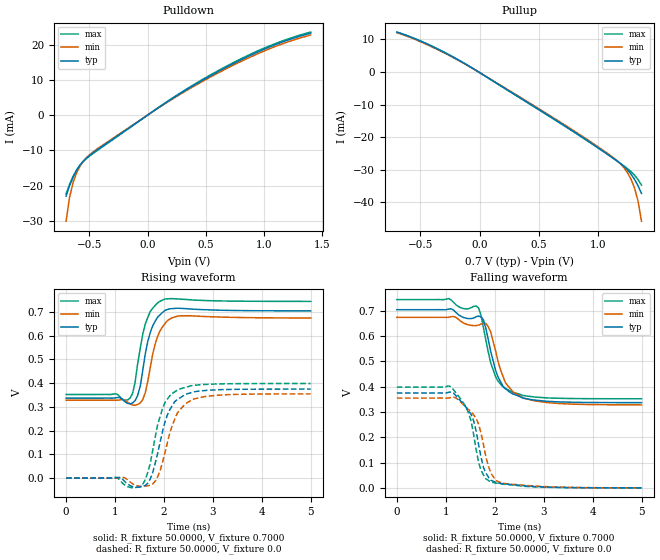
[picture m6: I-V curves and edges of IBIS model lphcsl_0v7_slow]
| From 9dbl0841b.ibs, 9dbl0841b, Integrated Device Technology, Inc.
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|   Model lphcsl_0v7_slow
[Model]  lphcsl_0v7_slow
Model_type Output
Polarity   Non-Inverting
Vmeas =  0.4000V
Cref =   2.0000pF
Rref =   0.0
Vref =   0.4000V
C_comp   1.1000pF   1.0000pF   1.2000pF
[Temperature Range]   27.0000   70.0000   0.0
[Voltage Range]   0.7000V   0.6700V   0.7400V
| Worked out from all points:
|   slope of the pulldown table from 0 to 0.105 V, typ, clamps not added: 44.3 ohm
|   slope of the pullup table from 0 to 0.105 V, typ, clamps not added: 44.4 ohm
|   rising waveform, R_fixture 50.0000, V_fixture 0.7000: 20-80 % time 217ps typ, 229ps min, 222ps max; typ from 0.337 V to 0.704 V
|   rising waveform, R_fixture 50.0000, V_fixture 0.0: 20-80 % time 318ps typ, 335ps min, 287ps max; typ from 0 V to 0.375 V
|   falling waveform, R_fixture 50.0000, V_fixture 0.7000: 20-80 % time 328ps typ, 363ps min, 307ps max; typ from 0.704 V to 0.337 V
|   falling waveform, R_fixture 50.0000, V_fixture 0.0: 20-80 % time 301ps typ, 312ps min, 292ps max; typ from 0.375 V to 0 V
[Pulldown]
|Voltage   I(typ)   I(min)   I(max)
-700mV    -23mA      -30.13mA   -22.37mA
-670mV    -20.06mA   -23.34mA   -19.68mA
-640mV    -17.66mA   -19.18mA   -17.42mA
-610mV    -15.72mA   -16.44mA   -15.59mA
-550mV    -12.99mA   -13.03mA   -13.08mA
-460mV    -10.5mA    -10.25mA   -10.7mA
170mV     3.791mA    3.653mA    3.891mA
530mV     10.98mA    10.63mA    11.23mA
800mV     15.65mA    15.2mA     15.96mA
1.01V     18.83mA    18.32mA    19.15mA
1.22V     21.47mA    20.95mA    21.77mA
1.4V      23.24mA    22.71mA    23.56mA
[Pullup]
|Voltage   I(typ)   I(min)   I(max)
-700mV    12.25mA    12.08mA    12.21mA
-430mV    8.33mA     8.148mA    8.393mA
-130mV    2.65mA     2.576mA    2.694mA
650mV     -14.87mA   -14.61mA   -14.98mA
920mV     -21.21mA   -20.93mA   -21.31mA
1.13V     -26.43mA   -26.22mA   -26.47mA
1.22V     -28.93mA   -29.29mA   -28.78mA
1.25V     -29.97mA   -30.81mA   -29.61mA
1.28V     -31.24mA   -32.79mA   -30.52mA
1.31V     -32.85mA   -35.5mA    -31.6mA
1.34V     -34.83mA   -39.47mA   -32.96mA
1.37V     -37.24mA   -45.78mA   -34.69mA
[Ramp]
| variable   typ   min   max
dV/dt_r  0.2250/0.3179n   0.2129/0.3346n   0.2390/0.2872n
dV/dt_f  0.2205/0.3282n   0.2077/0.3631n   0.2353/0.3071n
R_load = 50.0000
[Rising Waveform]
R_fixture= 50.0000
V_fixture= 0.7000
V_fixture_min= 0.6700
V_fixture_max= 0.7400
|time   V(typ)   V(min)   V(max)
0s        336.9mV    328mV      352.2mV
1.31ns    313.4mV    312mV      337.7mV
1.41ns    326.3mV    306.7mV    403mV
1.46ns    345.9mV    309.5mV    477.8mV
1.52ns    390.5mV    317.4mV    551.5mV
1.62ns    524.3mV    360.4mV    649.1mV
1.82ns    660.4mV    564.2mV    727.1mV
2.02ns    706.2mV    650.1mV    754.3mV
2.32ns    715.4mV    683.5mV    754.2mV
5ns       704.5mV    674.4mV    744.4mV
[Rising Waveform]
R_fixture= 50.0000
V_fixture= 0.0
V_fixture_min= 0.0
V_fixture_max= 0.0
|time   V(typ)   V(min)   V(max)
0s        629.4nV    0V         772.1nV
1.01ns    763.7uV    -128.1uV   3.786mV
1.16ns    -6.221mV   3.271mV    -22.91mV
1.52ns    -37.48mV   -34.9mV    -34.03mV
1.72ns    -3.843mV   -29.44mV   60.87mV
1.87ns    102.7mV    4.716mV    223.1mV
2.07ns    266.2mV    148.5mV    332.2mV
2.32ns    336.8mV    286.3mV    375.1mV
2.88ns    369.7mV    344.6mV    394.9mV
5ns       375mV      354.8mV    398.4mV
[Falling Waveform]
R_fixture= 50.0000
V_fixture= 0.7000
V_fixture_min= 0.6700
V_fixture_max= 0.7400
|time   V(typ)   V(min)   V(max)
0s        704.4mV    674.2mV    744.4mV
1.06ns    706.9mV    674.6mV    748.3mV
1.67ns    679.1mV    643.5mV    711.7mV
1.77ns    664mV      650.4mV    633.2mV
1.87ns    584.3mV    636.4mV    535.6mV
2.02ns    463.8mV    539.8mV    438.9mV
2.22ns    391.6mV    415.2mV    393.1mV
2.37ns    371.4mV    380.4mV    377.5mV
3.08ns    342.2mV    337mV      355.5mV
5ns       336.9mV    328.1mV    352.2mV
[Falling Waveform]
R_fixture= 50.0000
V_fixture= 0.0
V_fixture_min= 0.0
V_fixture_max= 0.0
|time   V(typ)   V(min)   V(max)
0s        375mV      355mV      398.5mV
1.11ns    379.3mV    357.5mV    398.6mV
1.46ns    306.2mV    310mV      298.9mV
1.52ns    289.6mV    299.9mV    262.6mV
1.62ns    225.3mV    274.2mV    152mV
1.77ns    81mV       171.7mV    51.27mV
1.92ns    30.55mV    58.66mV    23.07mV
2.02ns    21.61mV    29.54mV    19mV
2.37ns    12.44mV    13.84mV    10.82mV
5ns       28.22uV    82.51uV    11.53uV
